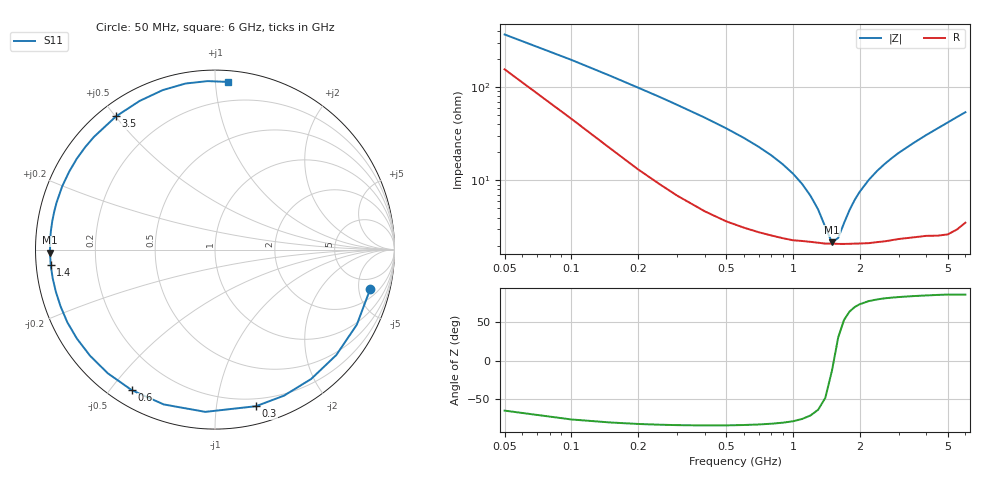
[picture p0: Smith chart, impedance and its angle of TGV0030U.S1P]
! SIEMENS Discrete & RF Semiconductors
! BAT64
! Si Schottky Diode in SOT23
! IF = 0.03 mA
! S-Parameters:  February  1997
# GHz  S  MA  R  50
!  f  S11
! GHz  MAG  ANG
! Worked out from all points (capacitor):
!   34 points, 50 MHz to 6 GHz, reference 50 ohm
!   read as one part to ground: C = 8.3 pF near 50 MHz
!   lowest |Z| = 2.16 ohm at 1.5 GHz (marker M1)
!   series resonance near 1.528 GHz, so ESL is about 1.3 nH
!   S11 on the Smith chart (normalised r, x): 50 MHz: 3.11, -6.66; 300 MHz: 0.14, -1.29; 600 MHz: 0.06, -0.57; 1.4 GHz: 0.04, -0.05; 3.5 GHz: 0.05, +0.50; 6 GHz: 0.07, +1.08
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0.05  0.8927 -14.1
0.1  0.894 -27.9
0.15  0.8955 -41.0
0.2  0.8981 -53.4
0.25  0.9 -64.7
0.3  0.9019 -75.3
0.4  0.9057 -93.4
0.5  0.9087 -108.3
0.6  0.9101 -120.6
0.7  0.9119 -130.9
0.8  0.9135 -139.6
0.9  0.9154 -147.2
1  0.917 -153.8
1.1  0.9167 -159.8
1.2  0.9173 -165.2
1.4  0.9195 -174.6
1.5  0.9192 -178.9
1.6  0.92 177.2
2  0.9208 163.5
2.4  0.9212 151.9
2.6  0.9216 146.7
3  0.9217 137.1
3.5  0.9247 126.6
4  0.9287 116.9
4.5  0.9351 108.2
5  0.9398 100.1
5.5  0.9396 92.5
6  0.9368 85.7
